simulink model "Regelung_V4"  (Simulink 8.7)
settings: Solver=ode45  StartTime=0.0  StopTime=25  MaxStep=0.5  MinStep=1e-2  RelTol=1e-3
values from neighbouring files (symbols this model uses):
  A = 1/n *     [ 0   n   0            0   ;                                0   0   b^2*p.g      0   ;                                0   0   0            n   ;                                0   0   mges*b*p.g   0 ]    [linPendelZR.m]    (also in initLinear.m = [; Aufgabe_VglEigenwerte.m = initLinear( l, mp, ms, 0, 0, g, pi ); Versuch2.m = initLinear( l, mp, ms, 0, 0, g, pi ); linPendelZR2.m = [0, 1, 0, 0)
  B = [0 a/n 0 b/n]'    [linPendelZR.m]    (also in initLinear.m = [0; 4; 0; 6/l]/(4*ms+mp); linPendelZR2.m = [0)
  K = 'Error'    [berechneLQR.m]    (also in simGUI.m = str2num(get(h.reglerK, 'String')))
  L = place(A.', C, obspoles).'    [berechneBeobachter.m]    (also in simGUI.m = berechneBeobachter(A, C, eigBeob); Versuch4.m = berechneBeobachter(A, C, eigBeob))
  stPendel = ladePendel()    [simGUI.m]    (also in systemPendel_V3.m = block.DialogPrm(1).Data; Versuch4.m; Versuch3.m; systemPendel_V5.m = block.DialogPrm(1).Data)
  wahl = 1    [simGUI.m]
  x0 = [x1_0 x2_0 x3_0 x4_0]    [simGUI.m]    (also in systemPendel_V3.m = block.DialogPrm(2).Data; Versuch4.m = [0.5 0 0 0]; Versuch3.m = [0.5 0 1*AP 0]; systemPendel_V5.m = block.DialogPrm(2).Data)
  xArbeitspunkt = [0, 0, AP, 0]    [runPendel.m]
undefined symbols (not defined in the file or in its folder): x0_obs

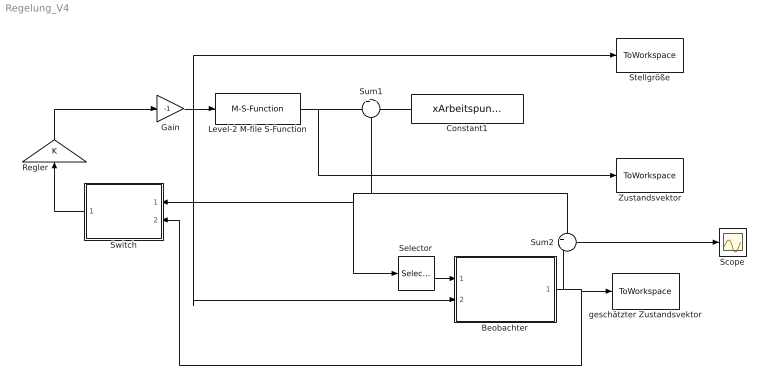
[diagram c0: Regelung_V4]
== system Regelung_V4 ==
  Beobachter : Subsystem
  Constant1 : Constant  Value=xArbeitspunkt
  Gain : Gain  Gain=-1
  Level-2 M-file S-Function : M-S-Function  FunctionName=systemPendel_V3  Parameters=stPendel,x0
  Regler : Gain  Gain=K  Multiplication=Matrix(K*u)
  Scope : Scope
  Selector : Selector  InputPortWidth=4  IndexOptions=Index vector (dialog)  Indices=[1 3]  OutputSizes=1
  Stellgröße : ToWorkspace  VariableName=vStell  SampleTime=-1
  Sum1 : Sum  Inputs=+|-
  Sum2 : Sum  Inputs=+|-
  Switch : Subsystem
  Zustandsvektor : ToWorkspace  VariableName=mZustand  SampleTime=-1
  geschätzter Zustandsvektor : ToWorkspace  VariableName=mBeobachter  SampleTime=-1
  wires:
  Regler/1 -> Gain/1
  Constant1/1 -> Sum1/2
  Sum1/1 -> Sum2/1, Switch/1(Zustand), Selector/1
  Gain/1 -> Level-2 M-file S-Function/1, Beobachter/2(u), Stellgröße/1
  Switch/1(zu Regler) -> Regler/1
  Beobachter/1(x_obs) -> geschätzter Zustandsvektor/1, Switch/2(Beob), Sum2/2
  Selector/1 -> Beobachter/1(y)
  Level-2 M-file S-Function/1 -> Sum1/1, Zustandsvektor/1
  Sum2/1 -> Scope/1

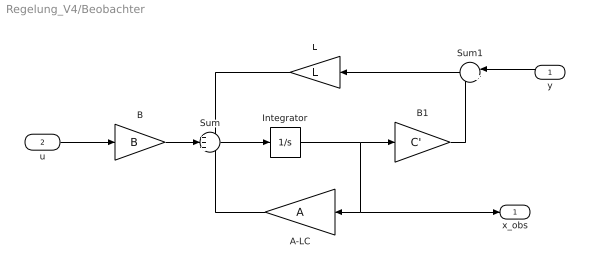
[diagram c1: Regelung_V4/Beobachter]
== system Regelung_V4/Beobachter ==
  y : Inport
  u : Inport  Port=2
  A-LC : Gain  Gain=A  Multiplication=Matrix(K*u)
  B : Gain  Gain=B  Multiplication=Matrix(K*u)
  B1 : Gain  Gain=C'  Multiplication=Matrix(K*u)
  Integrator : Integrator  InitialCondition=x0_obs
  L : Gain  Gain=L  Multiplication=Matrix(K*u)
  Sum : Sum  Inputs=+++
  Sum1 : Sum  Inputs=|+-
  x_obs : Outport
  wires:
  u/1 -> B/1
  B/1 -> Sum/2
  Sum/1 -> Integrator/1
  Integrator/1 -> B1/1, A-LC/1, x_obs/1
  A-LC/1 -> Sum/3
  L/1 -> Sum/1
  Sum1/1 -> L/1
  y/1 -> Sum1/1
  B1/1 -> Sum1/2

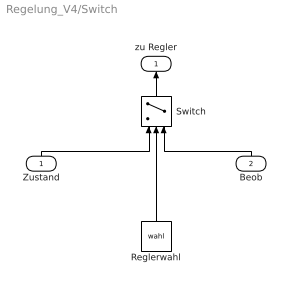
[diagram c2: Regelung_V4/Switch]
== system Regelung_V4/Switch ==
  Zustand : Inport
  Beob : Inport  Port=2
  Reglerwahl : Constant  Value=wahl
  Switch : Switch
  zu Regler : Outport
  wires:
  Reglerwahl/1 -> Switch/2
  Switch/1 -> zu Regler/1
  Zustand/1 -> Switch/1
  Beob/1 -> Switch/3
